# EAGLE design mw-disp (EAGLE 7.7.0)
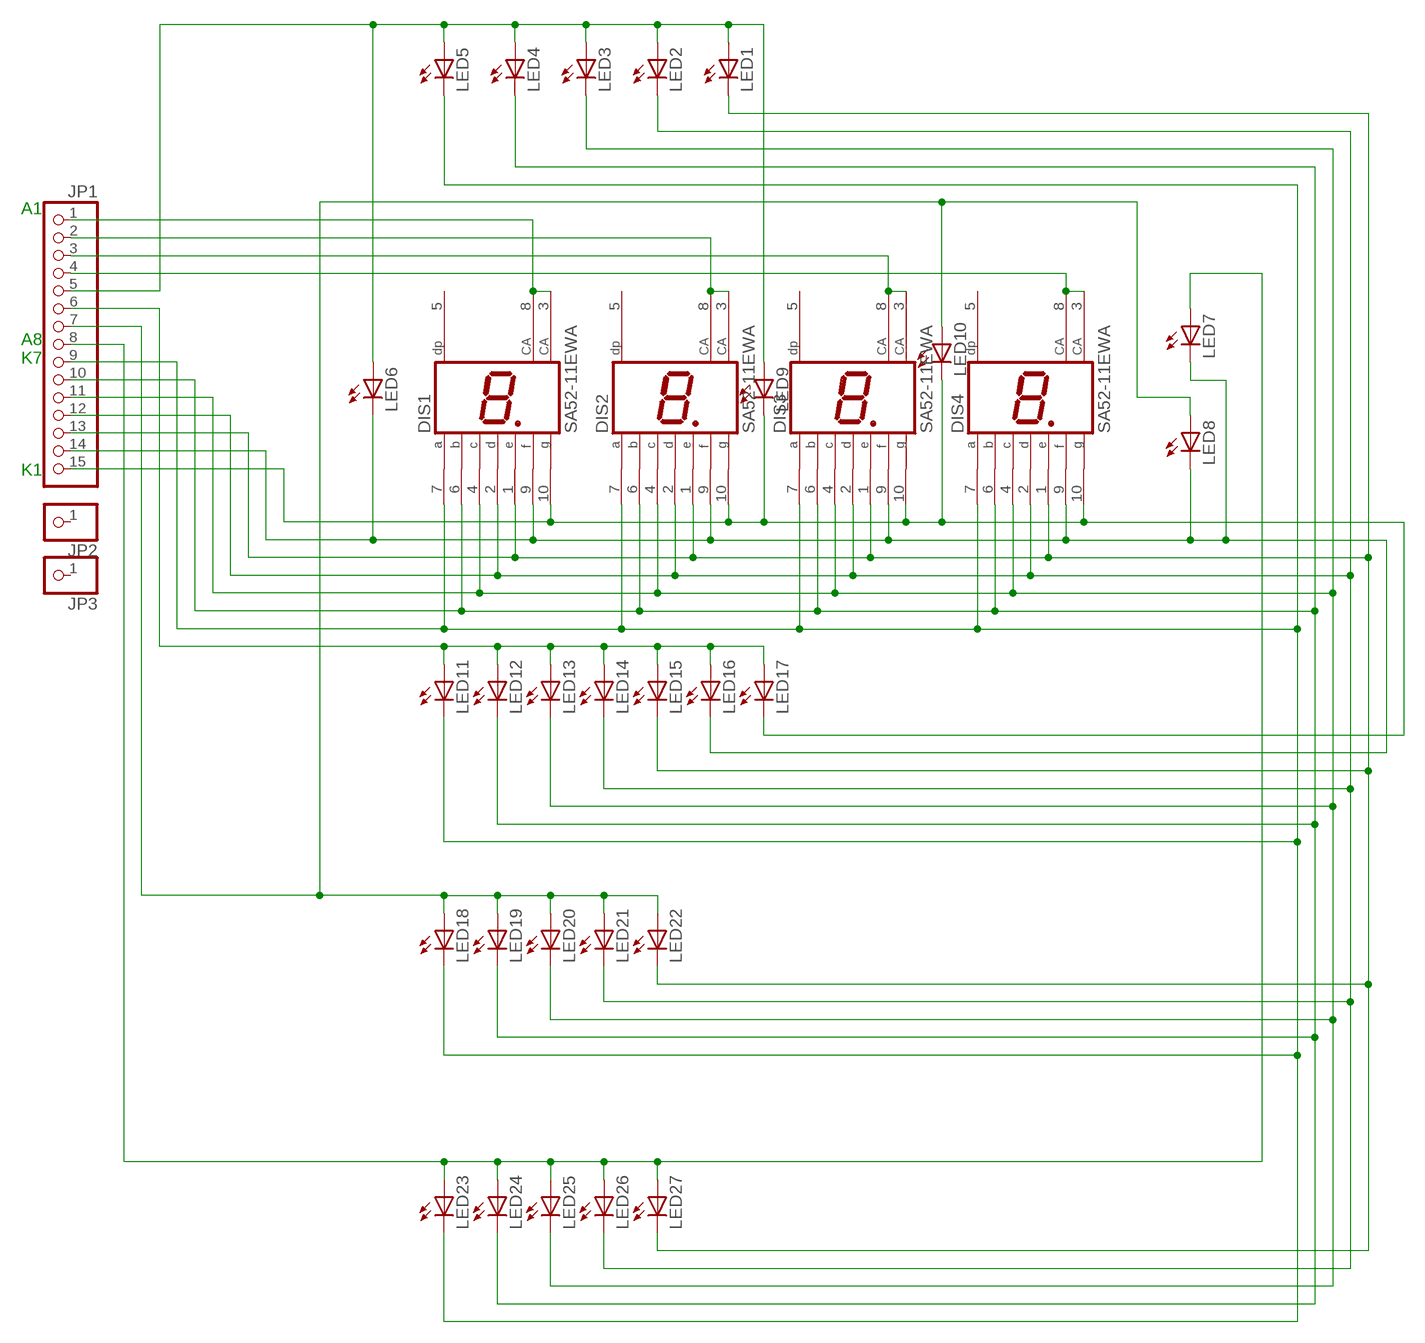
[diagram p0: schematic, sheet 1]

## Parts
DIS1  SA52-11EWA  HD-H101  [HDSP-M]
DIS2  SA52-11EWA  HD-H101  [HDSP-M]
DIS3  SA52-11EWA  HD-H101  [HDSP-M]
DIS4  SA52-11EWA  HD-H101  [HDSP-M]
JP1  PINHD-1X15  [1X15]
JP2  PINHD-1X1  [1X01]
JP3  PINHD-1X1  [1X01]
LED1  LED3MM  [LED3MM]
LED2  LED3MM  [LED3MM]
LED3  LED3MM  [LED3MM]
LED4  LED3MM  [LED3MM]
LED5  LED3MM  [LED3MM]
LED6  LED3MM  [LED3MM]
LED7  LED3MM  [LED3MM]
LED8  LED3MM  [LED3MM]
LED9  LED3MM  [LED3MM]
LED10  LED3MM  [LED3MM]
LED11  LED3MM  [LED3MM]
LED12  LED3MM  [LED3MM]
LED13  LED3MM  [LED3MM]
LED14  LED3MM  [LED3MM]
LED15  LED3MM  [LED3MM]
LED16  LED3MM  [LED3MM]
LED17  LED3MM  [LED3MM]
LED18  LED3MM  [LED3MM]
LED19  LED3MM  [LED3MM]
LED20  LED3MM  [LED3MM]
LED21  LED3MM  [LED3MM]
LED22  LED3MM  [LED3MM]
LED23  LED3MM  [LED3MM]
LED24  LED3MM  [LED3MM]
LED25  LED3MM  [LED3MM]
LED26  LED3MM  [LED3MM]
LED27  LED3MM  [LED3MM]

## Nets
N$1: JP1.5 LED1.A LED2.A LED3.A LED4.A LED5.A LED6.A LED9.A
N$2: DIS1.3(CA) DIS1.8(CA) JP1.1
N$3: DIS2.3(CA) DIS2.8(CA) JP1.2
N$4: DIS3.3(CA) DIS3.8(CA) JP1.3
N$5: DIS4.3(CA) DIS4.8(CA) JP1.4
N$7: JP1.6 LED11.A LED12.A LED13.A LED14.A LED15.A LED16.A LED17.A
N$8: JP1.7 LED8.A LED10.A LED18.A LED19.A LED20.A LED21.A LED22.A
N$11: JP1.8 LED7.A LED23.A LED24.A LED25.A LED26.A LED27.A
N$12: DIS1.10(G) DIS2.10(G) DIS3.10(G) DIS4.10(G) JP1.15 LED9.K(C) LED10.K(C) LED17.K(C)
N$13: DIS1.9(F) DIS2.9(F) DIS3.9(F) DIS4.9(F) JP1.14 LED6.K(C) LED7.K(C) LED8.K(C) LED16.K(C)
N$14: DIS1.1(E) DIS2.1(E) DIS3.1(E) DIS4.1(E) JP1.13 LED1.K(C) LED15.K(C) LED22.K(C) LED27.K(C)
N$15: DIS1.2(D) DIS2.2(D) DIS3.2(D) DIS4.2(D) JP1.12 LED2.K(C) LED14.K(C) LED21.K(C) LED26.K(C)
N$16: DIS1.4(C) DIS2.4(C) DIS3.4(C) DIS4.4(C) JP1.11 LED3.K(C) LED13.K(C) LED20.K(C) LED25.K(C)
N$17: DIS1.6(B) DIS2.6(B) DIS3.6(B) DIS4.6(B) JP1.10 LED4.K(C) LED12.K(C) LED19.K(C) LED24.K(C)
N$18: DIS1.7(A) DIS2.7(A) DIS3.7(A) DIS4.7(A) JP1.9 LED5.K(C) LED11.K(C) LED18.K(C) LED23.K(C)
Unconnected: DIS1.5(DP) DIS2.5(DP) DIS3.5(DP) DIS4.5(DP) JP2.1 JP3.1

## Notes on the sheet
- A1
  
  
  
  
  
  
  A8
  K7
  
  
  
  
  
  K1

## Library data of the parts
DIS1-DIS4 = display-hp:HD-H101: LED DISPLAY 1-character 7 segment, decimal point right
JP1 = pinhead:PINHD-1X15: PIN HEADER
JP2 JP3 = pinhead:PINHD-1X1: PIN HEADER
LED1-LED27 = led:LED: LED

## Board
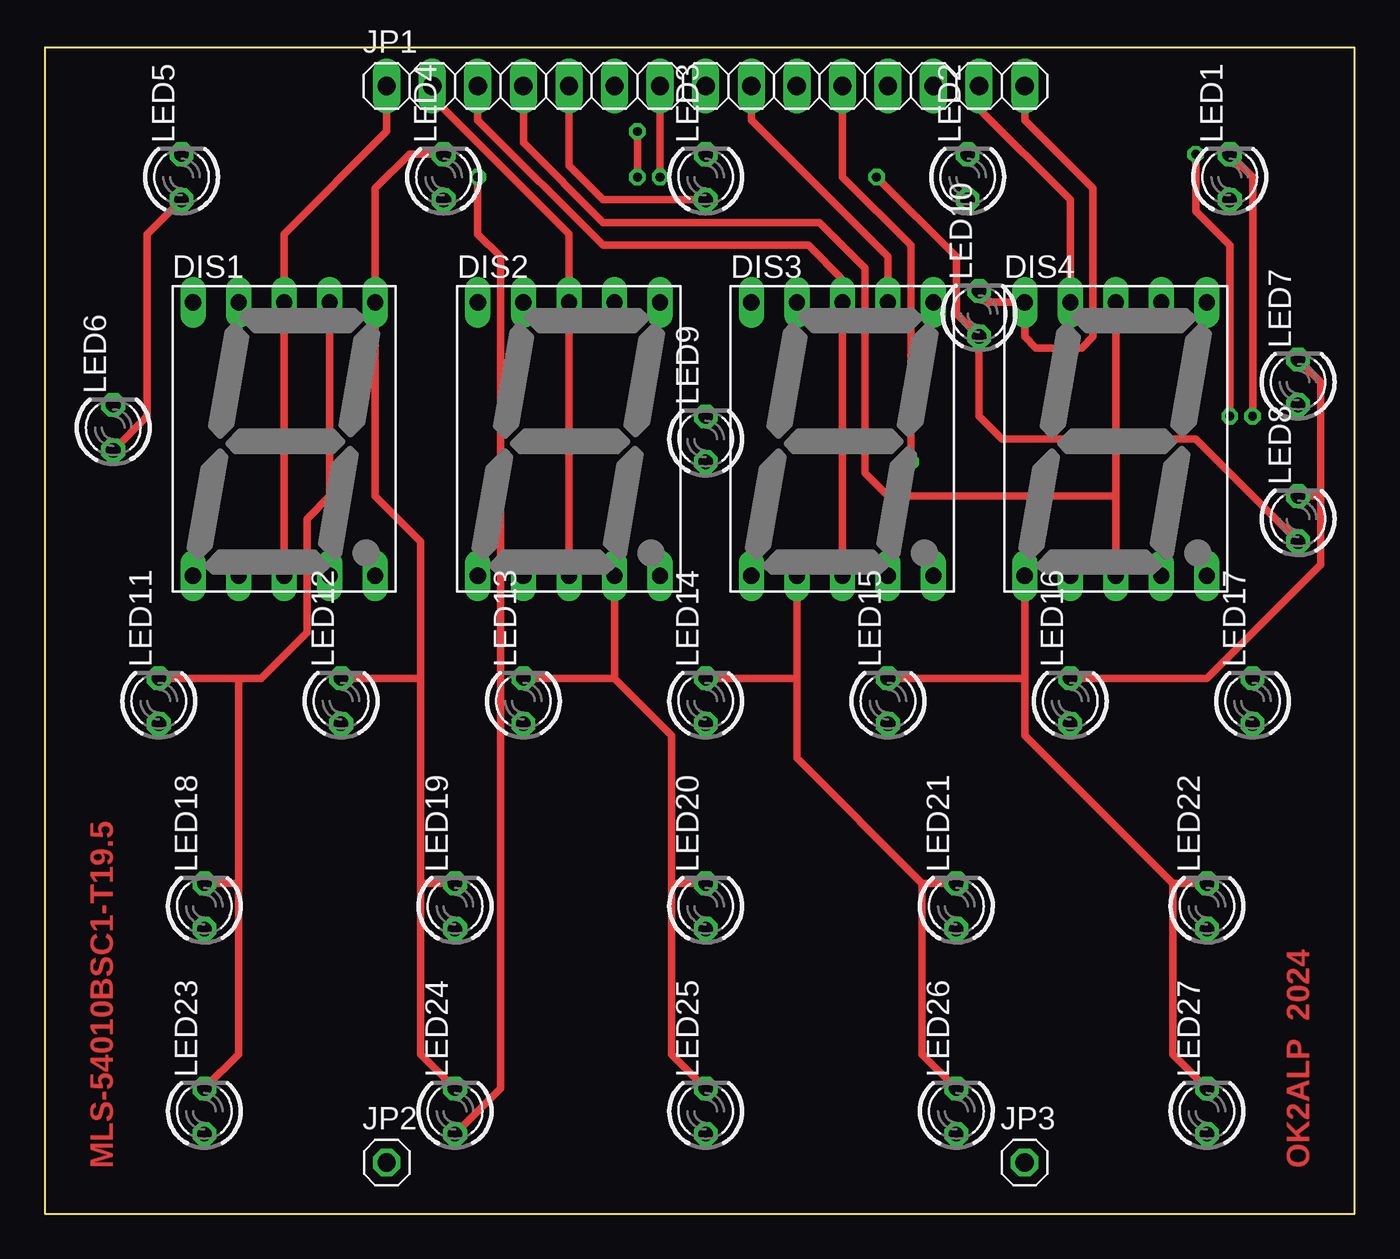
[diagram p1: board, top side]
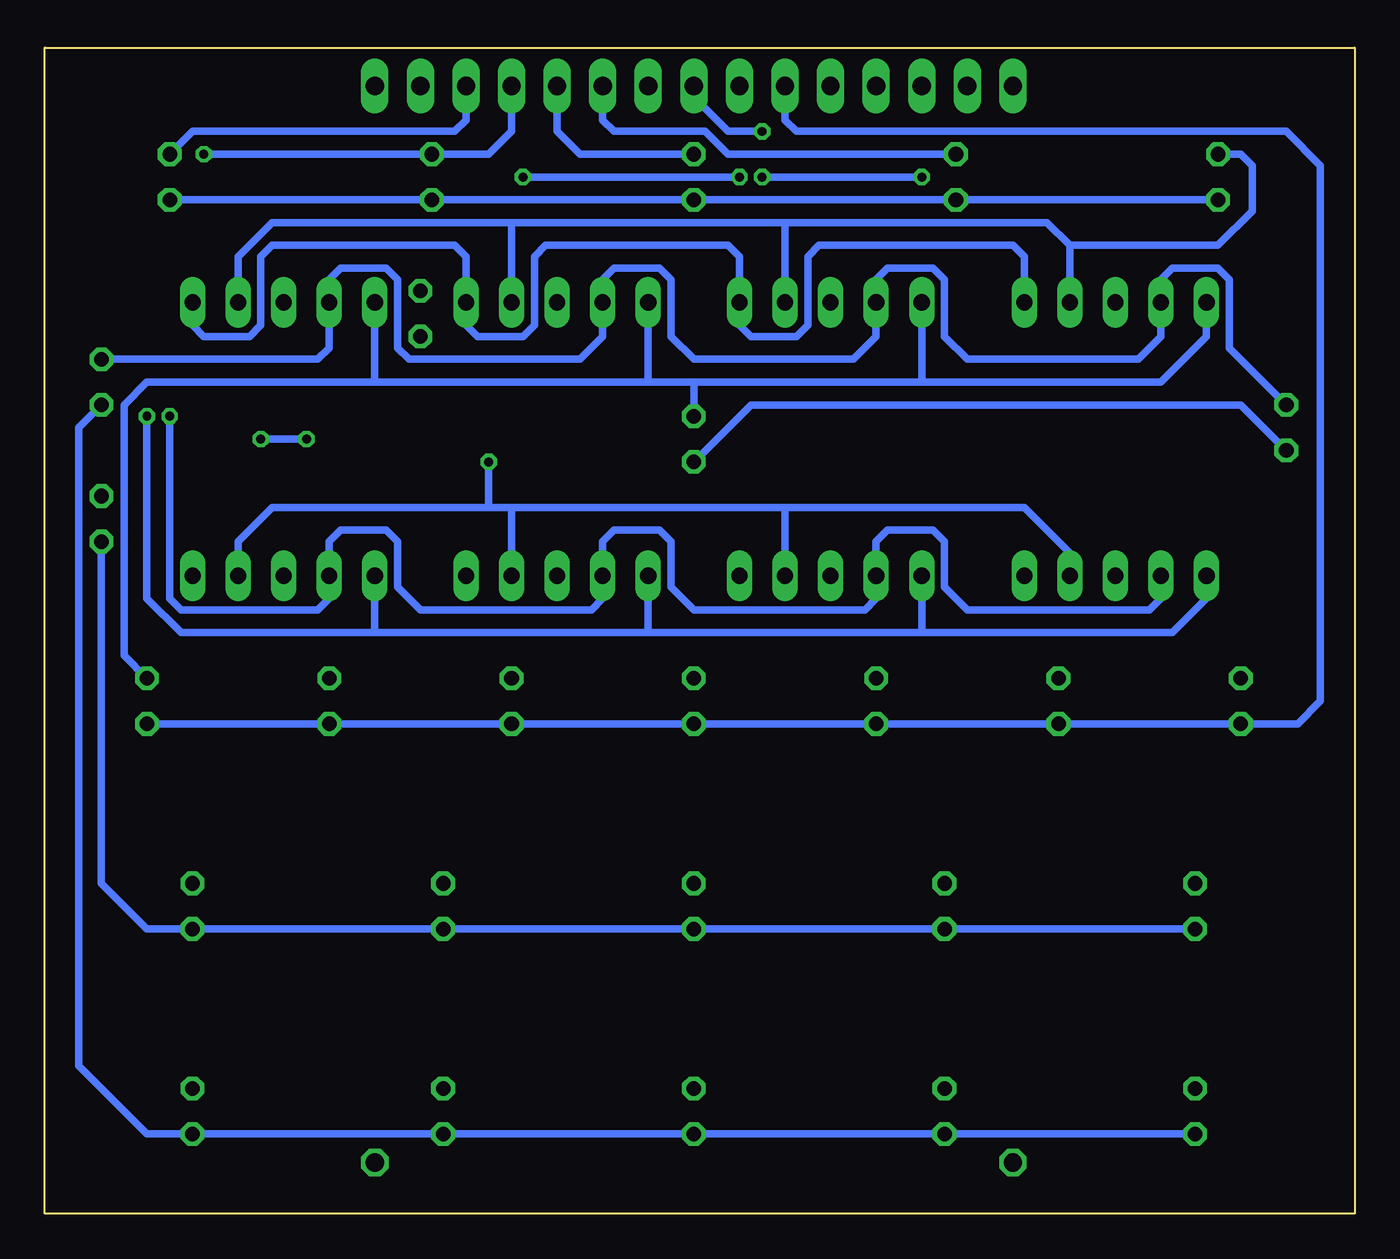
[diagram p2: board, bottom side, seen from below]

Size 73 x 65 mm. Coordinates in mm from the lower left corner, seen from the top.
Outline: 0,0 73,0 73,65 0,65 0,0
Copper layers (1*16): Top 0.035mm / dielectric 1.5mm / Bottom 0.035mm
Design rules "default *": minimum track width 10mil, minimum drill 24mil, track to track 8mil, track to pad 8mil, pad to pad 8mil, via to via 8mil, smd to smd 8mil, copper to edge 40mil, drill to drill 8mil, minimum pad ring 10mil, minimum via ring 8mil, stop-mask expansion 4mil, vias tented up to drill 0.5mm, thermal gap 10mil

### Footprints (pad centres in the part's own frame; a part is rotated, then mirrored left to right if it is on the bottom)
HDSP-M = drill 0.9 long: 1 -5.08,-7.62; 2 -2.54,-7.62; 3 0,-7.62; 4 2.54,-7.62; 5 5.08,-7.62; 6 5.08,7.62; 7 2.54,7.62; 8 0,7.62; 9 -2.54,7.62; 10 -5.08,7.62
1X15 = drill 1.016 long: 1 -17.78,0; 2 -15.24,0; 3 -12.7,0; 4 -10.16,0; 5 -7.62,0; 6 -5.08,0; 7 -2.54,0; 8 0,0; 9 2.54,0; 10 5.08,0; 11 7.62,0; 12 10.16,0; 13 12.7,0; 14 15.24,0; 15 17.78,0
1X01 = drill 1.016 octagon: 1 0,0
LED3MM = drill 0.813 octagon: A -1.27,0; K 1.27,0

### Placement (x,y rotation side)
DIS1  13.34,43.18 0 top
DIS2  29.21,43.18 0 top
DIS3  44.45,43.18 0 top
DIS4  59.69,43.18 0 top
JP1  36.83,62.87 0 top
JP2  19.05,2.86 0 top
JP3  54.61,2.86 0 top
LED1  66.04,57.78 90 top
LED2  51.44,57.78 90 top
LED3  36.83,57.78 90 top
LED4  22.23,57.78 90 top
LED5  7.62,57.78 90 top
LED6  3.81,43.81 90 top
LED7  69.85,46.35 90 top
LED8  69.85,38.73 90 top
LED9  36.83,43.18 90 top
LED10  52.07,50.16 90 top
LED11  6.35,28.57 90 top
LED12  16.51,28.57 90 top
LED13  26.67,28.57 90 top
LED14  36.83,28.57 90 top
LED15  46.99,28.57 90 top
LED16  57.15,28.57 90 top
LED17  67.31,28.57 90 top
LED18  8.89,17.14 90 top
LED19  22.86,17.14 90 top
LED20  36.83,17.14 90 top
LED21  50.8,17.14 90 top
LED22  64.77,17.14 90 top
LED23  8.89,5.71 90 top
LED24  22.86,5.71 90 top
LED25  36.83,5.71 90 top
LED26  50.8,5.71 90 top
LED27  64.77,5.71 90 top

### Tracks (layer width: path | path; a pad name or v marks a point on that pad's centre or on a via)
N$1
  Top 0.406: JP1.5 29.21,58.42 31.11,56.52 LED3.A | LED5.A 5.71,54.61 5.71,44.45 LED6.A
  Bottom 0.406: LED5.A LED4.A LED3.A LED2.A LED1.A | LED9.A 33.66,45.09 6.35,45.09 LED6.A
N$2
  Top 0.406: DIS1.3 DIS1.8 13.34,54.61 19.05,60.33 JP1.1
N$3
  Top 0.406: DIS2.3 DIS2.8 29.21,54.61 21.59,62.23 JP1.2
N$4
  Top 0.406: DIS3.3 DIS3.8 44.45,52.07 42.55,53.98 31.11,53.98 24.13,60.96 JP1.3
N$5
  Top 0.406: DIS4.3 59.69,40.01 | 59.69,40.01 DIS4.8 | JP1.4 26.67,59.69 31.11,55.24 43.18,55.24 45.72,52.7 45.72,41.27 46.99,40.01 59.69,40.01
N$7
  Bottom 0.406: LED17.A LED16.A LED15.A LED14.A LED13.A LED12.A LED11.A 3.17,27.3 1.91,28.57 1.91,58.42 3.81,60.33 31.11,60.33 31.75,60.96 JP1.6
N$8  (via drill 0.5)
  Top 0.406: v58.42,43.18 53.34,43.18 52.07,44.45 LED10.A 50.8,50.16 50.8,53.34 v46.35,57.78 | v60.96,43.18 64.14,43.18 LED8.A | JP1.7 v34.29,57.78
  Bottom 0.406: LED18.A LED19.A LED20.A LED21.A LED22.A 67.31,15.88 69.85,18.41 LED8.A | v58.42,43.18 v60.96,43.18 | v46.35,57.78 v34.29,57.78
N$11  (via drill 0.5)
  Top 0.406: v33.02,60.33 v33.02,57.78 | v24.13,57.78 24.13,54.61 25.4,53.34 25.4,6.99 LED24.A
  Bottom 0.406: LED23.A LED24.A LED25.A LED26.A LED27.A 67.31,4.45 71.12,8.26 71.12,43.81 LED7.A | JP1.8 36.83,62.23 34.92,60.33 v33.02,60.33 | v33.02,57.78 v24.13,57.78
N$12
  Top 0.406: JP1.15 54.61,60.96 58.42,57.15 58.42,48.9 57.78,48.26 55.24,48.26 54.61,48.9 DIS4.10 52.7,50.8 LED10.K
  Bottom 0.406: 24.13,46.35 DIS2.10 | DIS3.10 39.37,46.35 | 39.37,46.35 36.83,46.35 | 36.83,46.35 24.13,46.35 | 24.13,46.35 10.79,46.35 8.26,48.9 DIS1.10 | DIS4.10 54.61,46.35 | 54.61,46.35 39.37,46.35 | LED9.K 36.83,46.35 | LED17.K 68.58,31.11 68.58,45.09 67.31,46.35 54.61,46.35
N$13
  Top 0.406: LED16.K 64.77,29.84 71.12,36.2 71.12,40.01 | LED7.K 71.12,46.35 71.12,40.01 | 71.12,40.01 LED8.K | JP1.14 52.07,61.59 57.15,56.52 DIS4.9
  Bottom 0.406: LED7.K 57.78,47.62 57.15,48.26 DIS4.9 57.15,52.07 56.52,52.7 53.98,52.7 53.34,52.07 53.34,48.26 52.7,47.62 43.18,47.62 41.91,48.9 DIS3.9 41.91,52.07 41.27,52.7 38.73,52.7 38.1,52.07 38.1,48.9 36.83,47.62 27.94,47.62 26.67,48.9 DIS2.9 26.67,52.07 26.04,52.7 23.5,52.7 22.86,52.07 22.86,48.9 21.59,47.62 12.06,47.62 10.79,48.9 DIS1.9 10.79,52.07 10.16,52.7 7.62,52.7 6.99,52.07 6.99,48.26 LED6.K
N$14  (via drill 0.5)
  Top 0.406: LED27.K 62.87,8.89 62.87,18.41 | 62.87,18.41 LED22.K | DIS4.1 54.61,29.84 | 54.61,29.84 54.61,26.67 62.87,18.41 | LED15.K 54.61,29.84 | v67.31,44.45 67.31,57.78 LED1.K
  Bottom 0.406: DIS1.1 8.26,34.29 10.16,32.38 24.13,32.38 | 24.13,32.38 DIS2.1 | DIS3.1 39.37,32.38 | 39.37,32.38 24.13,32.38 | 39.37,32.38 54.61,32.38 | 54.61,32.38 65.41,32.38 67.31,34.29 v67.31,44.45 | JP1.13 49.53,60.96 50.16,60.33 64.77,60.33 LED1.K | DIS4.1 54.61,32.38
N$15  (via drill 0.5)
  Top 0.406: LED26.K 48.9,8.89 48.9,18.41 | 48.9,18.41 41.91,25.4 41.91,29.84 | 41.91,29.84 DIS3.2 | LED21.K 48.9,18.41 | LED14.K 41.91,29.84 | v66.04,44.45 66.04,53.98 64.14,55.88 v64.14,59.05
  Bottom 0.406: DIS1.2 10.79,34.29 11.43,33.66 21.59,33.66 22.86,34.92 22.86,37.47 23.5,38.1 26.04,38.1 26.67,37.47 DIS2.2 26.67,34.29 27.3,33.66 36.83,33.66 38.1,34.92 38.1,37.47 38.73,38.1 41.27,38.1 41.91,37.47 DIS3.2 41.91,34.29 42.55,33.66 52.07,33.66 53.34,34.92 53.34,37.47 53.98,38.1 56.52,38.1 57.15,37.47 DIS4.2 57.15,34.29 57.78,33.66 65.41,33.66 66.04,34.29 v66.04,44.45 | JP1.12 46.99,60.33 48.26,59.05 LED2.K v64.14,59.05
N$16  (via drill 0.5)
  Top 0.406: LED25.K 34.92,8.89 34.92,18.41 | 34.92,18.41 LED20.K | LED13.K 31.75,29.84 | 31.75,29.84 34.92,26.67 34.92,18.41 | DIS2.4 31.75,29.84 | v48.26,41.91 48.26,53.98 44.45,57.78 JP1.11
  Bottom 0.406: DIS1.4 15.88,36.83 18.41,39.37 31.75,39.37 | 31.75,39.37 DIS2.4 | DIS4.4 62.23,37.47 60.33,39.37 48.26,39.37 | JP1.11 44.45,60.33 43.18,59.05 LED3.K | 31.75,39.37 46.99,39.37 | 46.99,39.37 48.26,39.37 | v48.26,41.91 48.26,39.37 | DIS3.4 46.99,39.37
N$17
  Top 0.406: LED24.K 20.95,8.89 20.95,18.41 | 20.95,18.41 LED19.K | LED12.K 20.95,29.84 | 20.95,29.84 20.95,18.41 | 20.95,29.84 20.95,37.47 18.41,40.01 DIS1.6 18.41,57.15 20.32,59.05 LED4.K
  Bottom 0.406: DIS1.6 18.41,53.34 19.05,53.98 29.84,53.98 30.48,53.34 30.48,49.53 31.11,48.9 33.66,48.9 34.29,49.53 DIS2.6 34.29,53.34 34.92,53.98 45.09,53.98 45.72,53.34 45.72,49.53 46.35,48.9 48.9,48.9 49.53,49.53 DIS3.6 49.53,53.34 50.16,53.98 60.33,53.98 60.96,53.34 60.96,49.53 61.59,48.9 64.14,48.9 64.77,49.53 DIS4.6 | JP1.10 41.91,60.96 41.27,60.33 36.2,60.33 34.92,59.05 LED4.K
N$18
  Top 0.406: LED23.K 10.79,8.89 10.79,18.41 | 10.79,18.41 LED18.K | LED11.K 10.79,29.84 | 10.79,29.84 10.79,18.41 | DIS1.7 15.88,40.01 14.61,38.73 14.61,32.38 12.06,29.84 10.79,29.84 | JP1.9 39.37,60.96 46.99,53.34 DIS3.7
  Bottom 0.406: 31.75,55.24 DIS2.7 | DIS3.7 46.99,55.24 | 46.99,55.24 31.75,55.24 | 31.75,55.24 17.14,55.24 15.88,53.98 | 15.88,53.98 DIS1.7 | 46.99,55.24 60.33,55.24 62.23,53.34 DIS4.7 | LED5.K 6.35,59.05 5.71,58.42 5.71,55.88 7.62,53.98 15.88,53.98

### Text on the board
Top: MLS-54010BSC1-T19.5 | OK2ALP 2024
200bmp: D:/Clipboard01c.bmp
